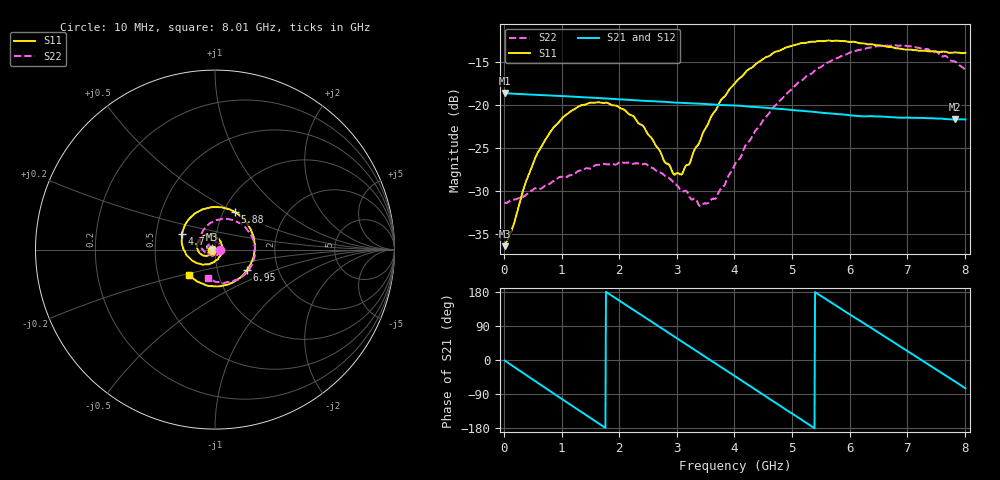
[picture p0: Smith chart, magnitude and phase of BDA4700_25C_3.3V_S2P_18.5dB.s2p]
!Agilent Technologies,E5071B,MY42404982,A.09.10
!Date: Mon Oct 20 18:10:49 2025
!Data & Calibration Information:
!Freq	S11:SOLT2(ON)	S21:SOLT2(ON)	S12:SOLT2(ON)	S22:SOLT2(ON)
# Hz S RI R 50
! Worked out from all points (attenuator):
!   801 points, 10 MHz to 8.01 GHz, reference 50 ohm
!   highest |S21| = -18.58 dB at 10 MHz (marker M1); lowest = -21.7 dB at 7.83 GHz (marker M2)
!   lowest |S11| = -36.4 dB at 10 MHz (marker M3), VSWR 1.03, Z = 48.5 - j0.118 ohm
!   |S11| at or under -10 dB: start of sweep to end of sweep
!   |S22| runs from -31.8 to -13.0 dB; largest |S21 - S12| = 0.0014
!   S11 on the Smith chart (normalised r, x): 10 MHz: 0.97, -0.00; 4.7 GHz: 0.68, +0.12; 5.88 GHz: 1.13, +0.50; 6.95 GHz: 1.39, -0.33; 8.01 GHz: 0.72, -0.21
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1e7  -0.015 -0.00122  0.1177 -0.00252  0.1177 -0.00263  0.027 -0.000844
6e8  -0.0414 -0.0344  0.0542 -0.1013  0.0542 -0.1013  0.0128 -0.0299
1.01e9  -0.0808 -0.0241  -0.0264 -0.11  -0.0264 -0.11  -0.0164 -0.0346
1.35e9  -0.0997 0.00948  -0.0827 -0.0747  -0.0828 -0.0748  -0.0381 -0.0171
2.07e9  -0.0476 0.0818  -0.0933 0.0545  -0.0933 0.0545  -0.029 0.0361
2.42e9  0.00199 0.0754  -0.0445 0.0965  -0.0446 0.0965  -0.00134 0.0453
2.68e9  0.0303 0.0469  0.00193 0.1052  0.00176 0.1051  0.017 0.0371
2.94e9  0.0392 0.00704  0.0468 0.0927  0.0468 0.0926  0.0284 0.0214
3.08e9  0.0359 -0.0161  0.0676 0.0781  0.0668 0.0786  0.0303 0.00965
3.4e9  0.00363 -0.0614  0.0972 0.0311  0.0973 0.0311  0.0212 -0.0147
3.53e9  -0.0173 -0.0744  0.1011 0.00852  0.1012 0.00839  0.0131 -0.0233
3.69e9  -0.0491 -0.0818  0.099 -0.0192  0.099 -0.0195  -0.00142 -0.029
4.01e9  -0.1167 -0.0671  0.0731 -0.0677  0.0731 -0.0675  -0.0356 -0.0277
4.7e9  -0.1852 0.0868  -0.0352 -0.0888  -0.0348 -0.0892  -0.0833 0.0535
5.35e9  -0.0594 0.2269  -0.0915 -0.00649  -0.0914 -0.00697  -0.0137 0.1532
5.88e9  0.1111 0.2093  -0.0594 0.0654  -0.0594 0.0652  0.1098 0.1608
6.27e9  0.1993 0.1123  -0.00791 0.0858  -0.00668 0.0856  0.1902 0.0972
6.68e9  0.217 -0.0293  0.049 0.0699  0.0491 0.0699  0.2215 -0.00845
6.95e9  0.1777 -0.1147  0.0738 0.0412  0.074 0.0407  0.2087 -0.0826
7.43e9  0.0353 -0.2029  0.08 -0.0257  0.08 -0.0259  0.1109 -0.1711
7.83e9  -0.0989 -0.1779  0.0453 -0.0691  0.0453 -0.0693  0.00394 -0.1799
8.01e9  -0.1468 -0.1393  0.0217 -0.0798  0.0221 -0.0798  -0.0382 -0.1569
